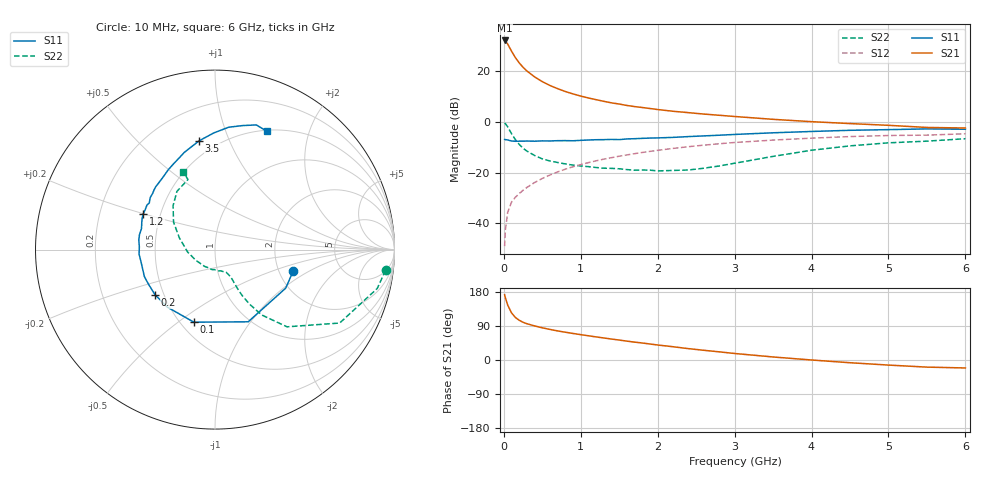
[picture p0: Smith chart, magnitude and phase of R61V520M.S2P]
! SIEMENS Small Signal Semiconductors
! BFR193
! Si NPN RF Bipolar Junction Transistor in SOT23
! VCE = 1.5 V  IC = 20 mA
! Common Emitter S-Parameters:  May  1996
# GHz  S  MA  R  50
!  f  S11  S21  S12  S22
! GHz  MAG  ANG  MAG  ANG  MAG  ANG  MAG  ANG
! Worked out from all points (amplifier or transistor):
!   36 points, 10 MHz to 6 GHz, reference 50 ohm
!   highest |S21| = 32.3 dB at 10 MHz (marker M1)
!   |S21| within 3 dB of that: start of sweep to 78.15 MHz
!   unconditionally stable (mu >= 1): 524 MHz to 2.099 GHz
!   at 250 MHz: K = 0.84, MSG = 24.3 dB, |S12| = -27.0 dB
!   at 1.4 GHz: K = 1.03, MAG = 9.8 dB, |S12| = -14.1 dB
!   at 6 GHz: K = 0.96, MSG = 1.1 dB, |S12| = -4.6 dB
!   S11 on the Smith chart (normalised r, x): 10 MHz: 2.40, -0.71; 100 MHz: 0.58, -0.57; 200 MHz: 0.45, -0.27; 1.2 GHz: 0.40, +0.20; 3.5 GHz: 0.40, +0.78; 6 GHz: 0.51, +1.41
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0.01  0.4521 -15.1  41.11 172.2  0.0035 82.5  0.9574 -6.9
0.02  0.4487 -28.6  39.96 164.4  0.0073 79.7  0.9294 -13.5
0.05  0.4427 -65.3  34.91 145.0  0.0163 70.6  0.8061 -30.5
0.1  0.4212 -106.2  25.27 124.3  0.0261 62.7  0.5883 -47.0
0.15  0.4161 -129.5  18.79 112.2  0.0325 60.4  0.4482 -54.4
0.2  0.418 -142.9  14.82 104.8  0.0384 62.3  0.3611 -57.6
0.25  0.4179 -152.7  12.09 99.5  0.0446 63.3  0.3027 -59.3
0.3  0.4212 -159.2  10.23 95.7  0.0509 64.9  0.2663 -59.9
0.4  0.4173 -169.6  7.82 89.9  0.0635 66.8  0.2182 -60.0
0.5  0.4238 -176.6  6.292 84.9  0.0766 67.9  0.1867 -60.0
0.6  0.4219 177.9  5.282 80.7  0.0895 68.4  0.1696 -60.7
0.7  0.428 172.7  4.567 76.7  0.1032 68.0  0.1583 -61.5
0.8  0.4289 168.8  4.015 73.3  0.1168 67.4  0.1485 -62.8
0.9  0.4259 164.1  3.594 70.0  0.1308 66.8  0.1402 -63.9
1.1  0.441 157.1  2.991 63.9  0.1574 65.1  0.1311 -69.5
1.2  0.4468 153.6  2.769 60.9  0.1709 64.2  0.1259 -72.5
1.6  0.4629 141.2  2.127 49.8  0.2235 59.2  0.1146 -87.9
2.2  0.4969 125.6  1.633 35.0  0.3006 50.8  0.1103 -122.2
3.5  0.6126 98.3  1.131 8.0  0.4395 30.6  0.2092 161.7
4.5  0.6861 83.6  0.932 -7.2  0.5155 16.2  0.3377 133.8
5.5  0.7317 71.7  0.781 -18.8  0.5508 2.0  0.4187 111.1
6  0.72 66.2  0.762 -21.0  0.5858 -2.2  0.4679 112.1
